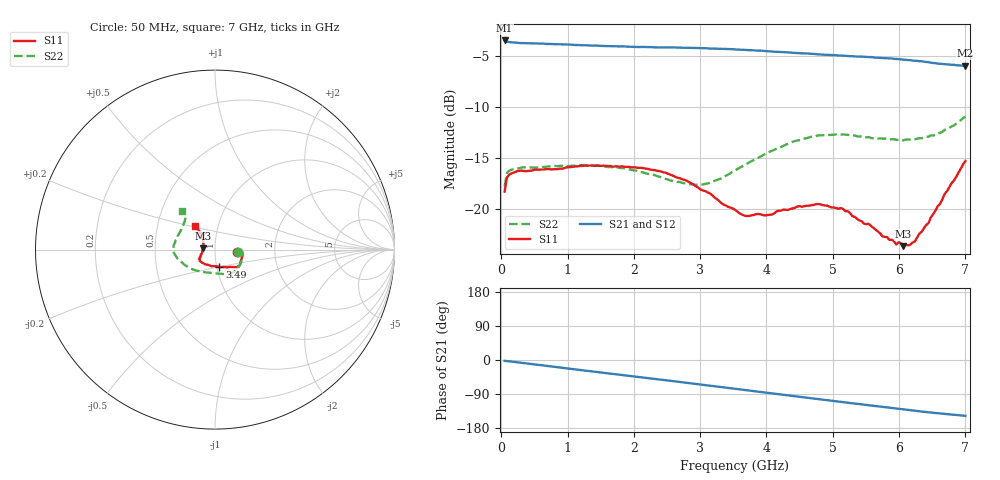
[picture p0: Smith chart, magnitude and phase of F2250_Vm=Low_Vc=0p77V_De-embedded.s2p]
! Integrated Device Technology
! Corporate Headquarters
! 6024 Silver Creek Valley Road
! San Jose, CA 95138  USA
! Phone:  1-408-284-8200
! Toll Free:  1-800-223-1366
! Webpage:  http://www.idt.com/
! Timing and RF Division
! 515 Groton Road, Suite 102
! Westford, MA 01886-6024
! Device:  F2250
! Description: Voltage Variable RF Attenuator
! Frequency:  50.0 -  6000.00 MHz
! Package:  3x3 mm Thin QFN Plastic Package: 16 pin
! Ports:  2 RF, 3 DC
!  Pin  1  = GND
!  Pin  2  = NC
!  Pin  3  = RF1  = Port 1
!  Pin  4  = NC
!  Pin  5  = GND
!  Pin  6  = GND
!  Pin  7  = GND
!  Pin  8  = GND
!  Pin  9  = NC
!  Pin 10  = RF2  = Port 2
!  Pin 11  = NC
!  Pin 12  = GND
!  Pin 13  = GND
!  Pin 14  = VCNTRL
!  Pin 15  = VDD
!  Pin 16  = VMODE
! Vcntrl:  0.770 Volts
! Vmode:  +0.000 Volts
! Vdd:  +3.30  Volts
! Current:  1.161 mA
! Data:  The device was measured on a the F2250 evaluation board which has
!  individual transmission lines to the RF pins.  Data was collected
!  using a calibrated network analyzer.  The evaluation board was
!  de-embedded using a TRL calibration technique.
!  The reference plane is the edge of the package pin.
! Misc:  SN 10
!  Action Tracker AT0258
! Date Measured:  2014-11-26
! Date:  2015-10-15  MJV
! Note:
!  Integrated Device Technology supplies this data as a sample of measured
!  data at the package pin for this product.  Your particular data for this
!  product may vary.
!  Data was taken at 25 degrees C.
!  Integrated Device Technology reserves the right to change this data at anytime.
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# GHz S dB R 50
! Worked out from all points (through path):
!   201 points, 50 MHz to 7 GHz, reference 50 ohm
!   highest |S21| = -3.43 dB at 50 MHz (marker M1); lowest = -5.9 dB at 7 GHz (marker M2)
!   group delay of S21, straight-line fit = 59.1 ps
!   lowest |S11| = -23.7 dB at 6.062 GHz (marker M3), VSWR 1.14, Z = 43.9 + j0.654 ohm
!   |S11| at or under -10 dB: start of sweep to end of sweep
!   |S22| runs from -17.8 to -10.9 dB; largest |S21 - S12| = 0.0015
!   S11 on the Smith chart (normalised r, x): 50 MHz: 1.27, -0.03; 3.49 GHz: 1.03, -0.20; 7 GHz: 0.78, +0.21
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0.05  -18.31 -5.4  -3.43 -2.3  -3.42 -2.3  -17.78 -6.7
0.08475  -16.93 -4.5  -3.55 -2.8  -3.56 -2.8  -16.48 -5.4
0.22375  -16.34 -7.0  -3.64 -5.6  -3.66 -5.6  -16.06 -9.6
1.2315  -15.78 -30.4  -3.91 -27.3  -3.91 -27.3  -15.70 -44.5
1.857  -15.87 -36.4  -4.02 -40.3  -4.03 -40.3  -16.02 -58.8
2.37825  -16.28 -39.3  -4.11 -51.2  -4.11 -51.2  -16.83 -71.1
2.79525  -17.23 -45.4  -4.16 -60.2  -4.16 -60.2  -17.52 -88.0
3.0385  -18.19 -52.5  -4.19 -65.5  -4.19 -65.5  -17.61 -101.8
3.49025  -19.97 -75.9  -4.29 -75.5  -4.29 -75.5  -16.35 -128.4
3.525  -20.10 -77.3  -4.31 -76.2  -4.31 -76.2  -16.24 -130.1
3.69875  -20.71 -90.0  -4.37 -80.1  -4.37 -80.1  -15.58 -138.7
3.97675  -20.65 -107.9  -4.49 -86.1  -4.48 -86.1  -14.62 -151.4
4.7065  -19.62 -141.5  -4.76 -101.8  -4.75 -101.8  -12.91 -173.9
5.1235  -19.93 -150.5  -4.92 -110.6  -4.91 -110.6  -12.71 176.5
5.471  -21.47 -158.2  -5.03 -117.8  -5.04 -117.8  -12.96 168.6
5.5405  -21.48 -160.7  -5.07 -119.3  -5.06 -119.4  -12.94 166.6
5.85325  -23.07 -172.7  -5.19 -125.8  -5.21 -125.8  -13.17 158.6
6.06175  -23.68 173.5  -5.32 -130.2  -5.32 -130.2  -13.27 152.3
6.2355  -23.23 156.5  -5.43 -133.7  -5.41 -133.8  -13.16 146.3
6.444  -21.42 141.9  -5.57 -137.9  -5.58 -138.0  -12.90 139.7
6.722  -18.28 131.0  -5.78 -142.8  -5.78 -142.8  -12.19 132.7
7  -15.30 129.3  -5.93 -147.3  -5.95 -147.3  -10.92 130.5
